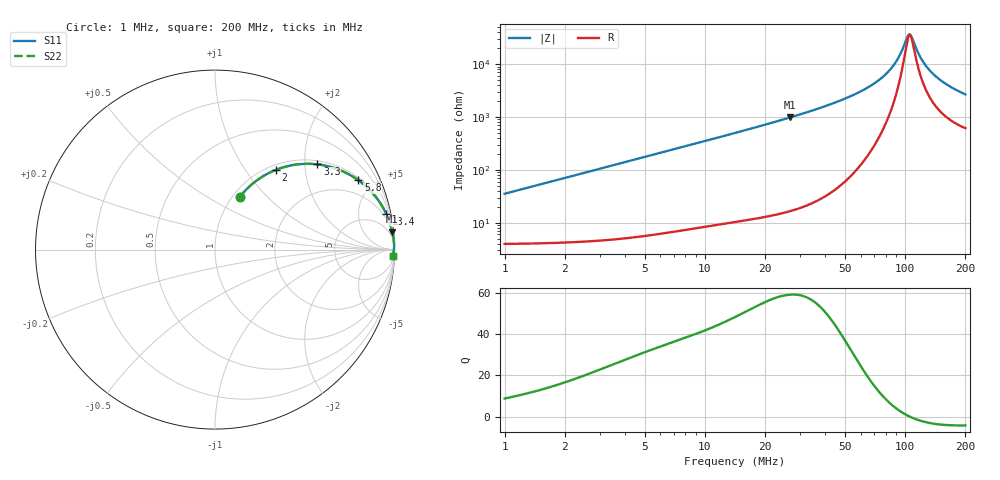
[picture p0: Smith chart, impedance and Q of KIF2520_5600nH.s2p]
!version-2
!date-12.2020
!Series
# MHz S RI R 50
!Freq ReS11 ImS11 ReS21 ImS21 ReS12 ImS12 ReS22 ImS22
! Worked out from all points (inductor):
!   1991 points, 1 MHz to 200 MHz, reference 50 ohm
!   read as one part in series: L = 5.59 uH near 1.9 MHz
!   highest Q = 59.2 at 26.7 MHz (marker M1), where L = 5.86 uH
!   self-resonance near 105.6 MHz
!   S11 on the Smith chart (normalised r, x): 1 MHz: 1.08, +0.70; 2 MHz: 1.08, +1.41; 3.3 MHz: 1.09, +2.32; 5.8 MHz: 1.12, +4.07; 13.4 MHz: 1.20, +9.44; 200 MHz: 13, -52
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1  0.137 0.2918  0.863 -0.2918  0.863 -0.2918  0.137 0.2918
2  0.3405 0.4448  0.6595 -0.4448  0.6595 -0.4448  0.3405 0.4448
3.3  0.5708 0.475  0.4292 -0.475  0.4292 -0.475  0.5708 0.475
4.5  0.7077 0.4382  0.2923 -0.4382  0.2923 -0.4382  0.7077 0.4382
5.8  0.7984 0.3865  0.2016 -0.3865  0.2016 -0.3865  0.7984 0.3865
8.7  0.8971 0.2915  0.1029 -0.2915  0.1029 -0.2915  0.8971 0.2915
13.4  0.9532 0.2009  0.0468 -0.2009  0.0468 -0.2009  0.9532 0.2009
19.3  0.977 0.1412  0.023 -0.1412  0.023 -0.1412  0.977 0.1412
26.7  0.9881 0.1002  0.0119 -0.1002  0.0119 -0.1002  0.9881 0.1002
34.2  0.993 0.0753  0.00705 -0.0753  0.00705 -0.0753  0.993 0.0753
67.4  0.9979 0.0254  0.00212 -0.0254  0.00212 -0.0254  0.9979 0.0254
78.6  0.998 0.0164  0.00204 -0.0164  0.00204 -0.0164  0.998 0.0164
87.3  0.9978 0.0105  0.00215 -0.0105  0.00215 -0.0105  0.9978 0.0105
94.1  0.9977 0.00631  0.00233 -0.00631  0.00233 -0.00631  0.9977 0.00631
100.5  0.9975 0.00271  0.00254 -0.00271  0.00254 -0.00271  0.9975 0.00271
103.8  0.9973 0.000958  0.00267 -0.000958  0.00267 -0.000958  0.9973 0.000958
106.4  0.9972 -0.000385  0.00278 0.000385  0.00278 0.000385  0.9972 -0.000385
119.5  0.9966 -0.00668  0.00342 0.00668  0.00342 0.00668  0.9966 -0.00668
133.7  0.9957 -0.0128  0.00427 0.0128  0.00427 0.0128  0.9957 -0.0128
148.2  0.9947 -0.0185  0.00528 0.0185  0.00528 0.0185  0.9947 -0.0185
166.9  0.9932 -0.0252  0.00676 0.0252  0.00676 0.0252  0.9932 -0.0252
200  0.9902 -0.0357  0.00982 0.0357  0.00982 0.0357  0.9902 -0.0357
